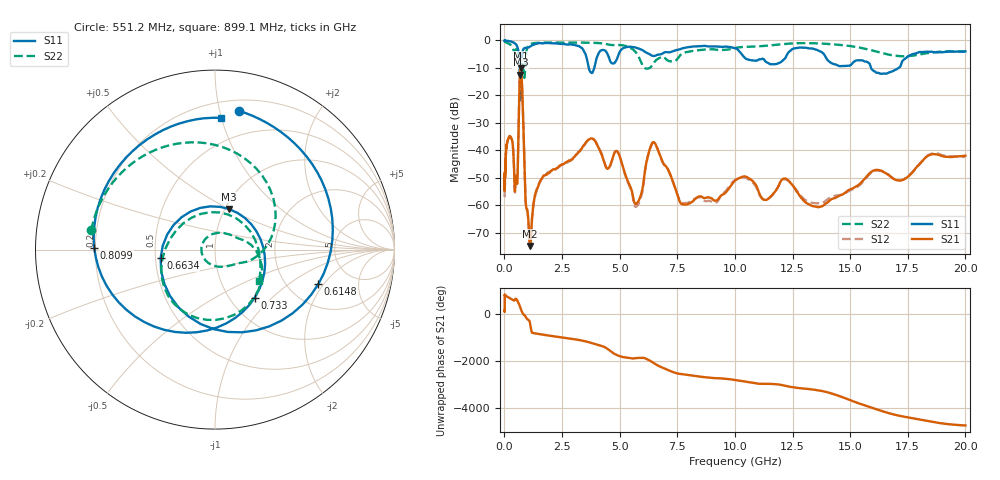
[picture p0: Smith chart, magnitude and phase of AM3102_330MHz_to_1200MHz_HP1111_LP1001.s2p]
! Date/Time: Tue, Sep 11, 2018 5:24 PM
! Network Analyzer: Agilent Technologies E8362B Rev: A.07.50.63
! Sweep from 0.010 to 20.000 GHz, 1601 Points, Sweep Type: LOG
! Power Supply: 4.949 V, 0.001 A
# Hz S DB R 50
!freq MagS11 AngS11 MagS21 AngS21 MagS12 AngS12 MagS22 AngS22
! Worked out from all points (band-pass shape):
!   1601 points, 10 MHz to 20 GHz, reference 50 ohm
!   highest |S21| = -10.08 dB at 705.6 MHz (marker M1); lowest = -74.8 dB at 1.124 GHz (marker M2)
!   |S21| within 3 dB of the highest: 669.5 MHz to 746.9 MHz (77.44 MHz wide, 10.9 % of centre)
!   lowest |S11| = -12.4 dB at 692.3 MHz (marker M3), VSWR 1.63, Z = 52.4 + j25.1 ohm
!   |S11| at or under -10 dB: 661.5 MHz to 725.8 MHz (64.36 MHz wide, 9.28 % of centre); 3.661 GHz to 3.9 GHz (238.5 MHz wide, 6.31 % of centre); 15.91 GHz to 17.1 GHz (1.195 GHz wide, 7.24 % of centre)
!   |S22| runs from -22.3 to -0.2 dB; largest |S21 - S12| = 0.0045
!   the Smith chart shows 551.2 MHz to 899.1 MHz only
!   S11 on the Smith chart (normalised r, x): 551.2 MHz: 0.29, +1.15; 614.8 MHz: 2.89, -1.78; 663.4 MHz: 0.53, -0.06; 733 MHz: 1.30, -0.79; 809.9 MHz: 0.20, +0.01; 899.1 MHz: 0.31, +1.00
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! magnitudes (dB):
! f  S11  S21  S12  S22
! 10 MHz  0.0  -48.4  -53.9  -0.3
! 35.55 MHz  -0.1  -46.2  -46.7  -0.5
! 126.4 MHz  -0.2  -36.9  -37.1  -0.9
! 337.9 MHz  -0.6  -36.5  -36.4  -2.4
! 447.2 MHz  -1.0  -54.1  -54.5  -3.8
! 551.2 MHz  -2.1  -52.3  -52.3  -3.1
! 614.8 MHz  -4.3  -30.6  -30.8  -4.5
! 663.4 MHz  -10.3  -14.3  -14.3  -9.9
! 692.3 MHz  -12.4  -10.5  -10.5  -20.3
! 705.6 MHz  -12.0  -10.1  -10.1  -22.2
! 733 MHz  -9.2  -11.4  -11.5  -19.6
! 809.9 MHz  -3.4  -27.0  -27.1  -8.5
! 899.1 MHz  -2.7  -54.3  -54.3  -10.4
! 1.124 GHz  -2.1  -74.8  -74.8  -1.3
! 1.59 GHz  -1.0  -50.6  -50.8  -0.8
! 3.793 GHz  -11.9  -35.7  -35.6  -0.8
! 5.652 GHz  -2.5  -59.3  -60.3  -3.8
! 6.457 GHz  -5.6  -37.0  -37.2  -8.5
! 7.882 GHz  -2.6  -59.8  -59.2  -4.3
! 10.38 GHz  -5.9  -49.5  -49.9  -2.4
! 13.68 GHz  -3.9  -60.6  -59.3  -1.1
! 20 GHz  -4.0  -42.0  -42.5  -4.0
